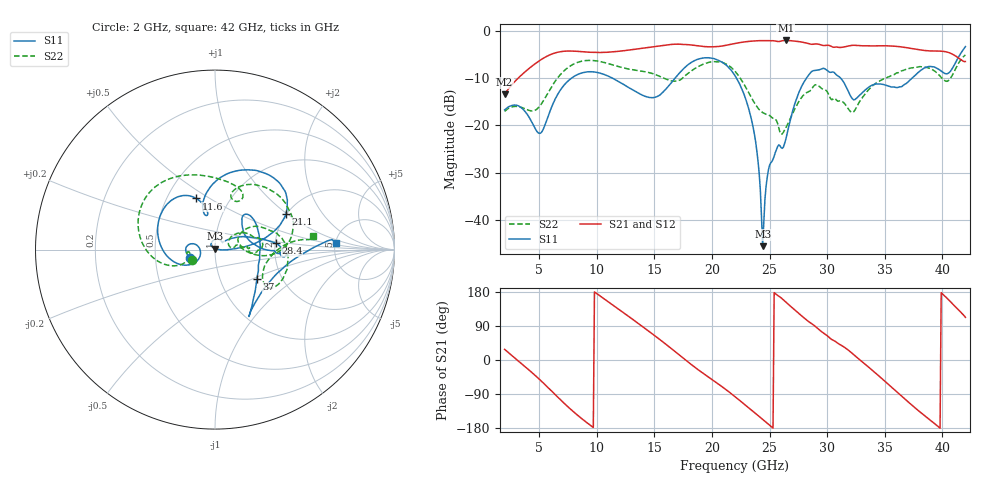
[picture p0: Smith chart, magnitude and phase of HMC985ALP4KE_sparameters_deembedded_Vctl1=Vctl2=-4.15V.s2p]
!s2p File: Measurements: S11, S21, S12, S22
# GHz S dB R 50.0
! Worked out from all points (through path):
!   401 points, 2 GHz to 42 GHz, reference 50 ohm
!   highest |S21| = -2.08 dB at 26.4 GHz (marker M1); lowest = -13.5 dB at 2 GHz (marker M2)
!   lowest |S11| = -45.6 dB at 24.4 GHz (marker M3), VSWR 1.01, Z = 50.2 + j0.475 ohm
!   |S11| at or under -10 dB: start of sweep to 7.837 GHz; 22.12 GHz to 28.22 GHz (6.1 GHz wide, 24.2 % of centre); 31.15 GHz to 37.39 GHz (6.245 GHz wide, 18.2 % of centre)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
!   |S22| runs from -21.9 to -5.1 dB; largest |S21 - S12| = 0.00058
!   S11 on the Smith chart (normalised r, x): 2 GHz: 0.75, -0.07; 11.6 GHz: 0.70, +0.44; 21.1 GHz: 1.98, +0.99; 28.4 GHz: 2.01, +0.16; 37 GHz: 1.50, -0.53; 42 GHz: 5.12, +0.64
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2  -16.76 -162.2  -13.46 28.1  -13.47 28.1  -17.08 -156.0
5.1  -21.70 -169.0  -6.24 -53.1  -6.25 -53.1  -15.81 -159.4
6.3  -14.93 -151.2  -4.78 -88.5  -4.79 -88.5  -11.02 -162.3
8.7  -8.95 149.9  -4.46 -154.9  -4.46 -154.9  -6.47 150.8
11.6  -10.36 110.1  -4.45 140.5  -4.45 140.5  -7.40 103.0
13.6  -13.20 101.5  -3.85 96.5  -3.85 96.6  -8.46 75.2
15.4  -13.74 106.6  -3.25 55.6  -3.25 55.6  -9.60 62.0
17.9  -7.25 79.5  -2.97 -4.6  -2.97 -4.6  -9.10 72.0
21.1  -7.05 26.9  -3.16 -75.4  -3.16 -75.4  -6.93 15.2
22  -9.51 16.5  -2.72 -96.7  -2.73 -96.7  -8.59 -0.1
23.6  -20.77 1.3  -2.20 -136.5  -2.20 -136.5  -14.94 -3.7
24.4  -45.56 63.7  -2.11 -156.7  -2.11 -156.7  -17.32 8.3
25  -28.46 127.7  -2.13 -172.0  -2.13 -172.0  -17.96 12.0
26.4  -23.05 41.6  -2.08 153.2  -2.08 153.2  -20.58 33.8
28.4  -9.37 6.0  -2.76 101.1  -2.76 101.1  -12.89 17.5
28.7  -8.57 1.0  -2.90 94.9  -2.90 94.9  -12.18 15.7
32.4  -14.60 30.2  -3.11 11.5  -3.11 11.5  -16.83 26.5
33.9  -11.53 48.1  -3.23 -26.7  -3.23 -26.7  -11.73 30.2
35.4  -11.76 17.7  -3.23 -66.7  -3.23 -66.6  -9.72 18.7
37  -10.89 -35.0  -3.65 -109.8  -3.65 -109.8  -8.07 4.0
39.8  -8.38 -56.1  -4.33 -179.9  -4.33 -179.9  -9.61 -34.5
42  -3.38 2.9  -6.54 112.6  -6.55 112.6  -5.13 7.7
